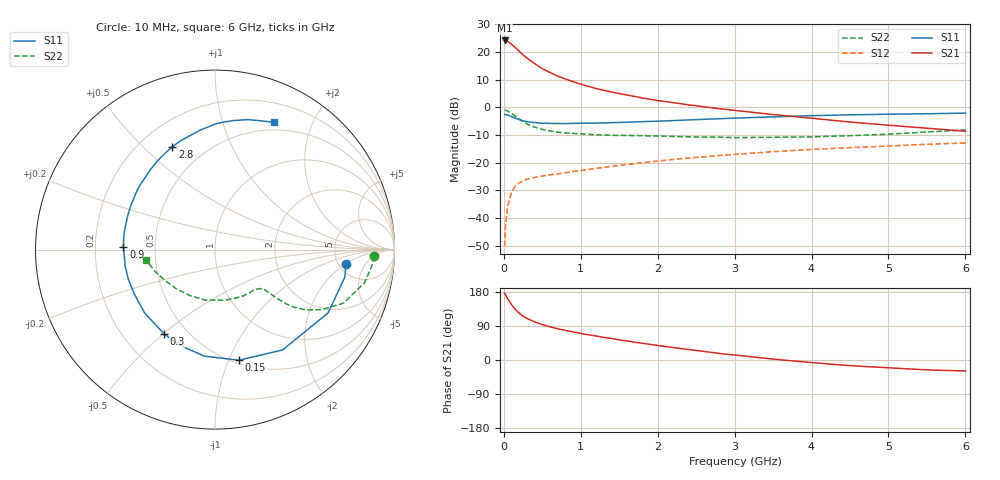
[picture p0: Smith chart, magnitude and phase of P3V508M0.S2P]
! SIEMENS Small Signal Semiconductors
! BFP181
! Si NPN RF Bipolar Junction Transistor in SOT143
! VCE = 0.5 V  IC = 8 mA
! Common Emitter S-Parameters:  March  1996
# GHz  S  MA  R  50
!  f  S11  S21  S12  S22
! GHz  MAG  ANG  MAG  ANG  MAG  ANG  MAG  ANG
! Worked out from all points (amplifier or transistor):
!   36 points, 10 MHz to 6 GHz, reference 50 ohm
!   highest |S21| = 24.1 dB at 10 MHz (marker M1)
!   |S21| within 3 dB of that: start of sweep to 165.1 MHz
!   unconditionally stable (mu >= 1): start of sweep to 10.12 MHz; 459.4 MHz to end of sweep
!   at 250 MHz: K = 0.61, MSG = 22.7 dB, |S12| = -26.6 dB
!   at 1.4 GHz: K = 1.95, MAG = 7.8 dB, |S12| = -21.3 dB
!   at 6 GHz: K = 2.00, MAG = -3.6 dB, |S12| = -12.9 dB
!   S11 on the Smith chart (normalised r, x): 10 MHz: 5.78, -2.06; 150 MHz: 0.53, -1.09; 300 MHz: 0.37, -0.50; 900 MHz: 0.32, +0.01; 2.8 GHz: 0.33, +0.62; 6 GHz: 0.41, +1.49
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0.01  0.7345 -6.4  16.03 176.4  0.0031 85.9  0.8855 -2.4
0.02  0.7391 -12.1  16.02 173.0  0.0067 80.3  0.8825 -5.1
0.05  0.7223 -29.2  15.46 161.7  0.0163 75.9  0.8534 -12.5
0.1  0.6742 -56.0  13.69 146.0  0.0292 61.7  0.7758 -22.6
0.15  0.6306 -77.7  11.87 133.3  0.0378 52.6  0.6829 -29.3
0.2  0.5966 -95.7  10.24 123.5  0.0432 46.8  0.6089 -33.5
0.25  0.5684 -110.1  8.793 115.8  0.0468 41.9  0.5464 -36.0
0.3  0.549 -121.2  7.711 110.0  0.0501 39.5  0.499 -37.3
0.4  0.5272 -138.3  6.111 100.5  0.0539 36.6  0.4378 -38.2
0.5  0.5134 -151.1  4.98 93.4  0.0573 35.0  0.3982 -38.5
0.6  0.5104 -161.1  4.235 87.5  0.0601 34.8  0.3721 -38.7
0.7  0.5089 -169.2  3.644 82.6  0.0625 35.3  0.3552 -39.0
0.9  0.5102 178.5  2.898 74.2  0.0692 36.1  0.3373 -40.3
1.1  0.5152 167.5  2.38 66.4  0.0754 37.1  0.3238 -42.6
1.5  0.5307 151.5  1.761 53.1  0.0888 38.1  0.3099 -48.6
1.8  0.5488 140.7  1.473 44.1  0.0993 37.9  0.3062 -54.5
2.2  0.5739 128.5  1.209 33.0  0.1138 36.5  0.2962 -63.7
2.8  0.6202 112.6  0.94 17.3  0.1343 33.2  0.2882 -79.3
3.5  0.669 97.5  0.737 2.4  0.1574 28.6  0.2865 -101.0
4.5  0.7271 81.7  0.54 -14.9  0.1861 20.1  0.306 -133.6
5.5  0.7623 70.2  0.418 -26.0  0.214 12.5  0.3571 -160.5
6  0.7818 65.0  0.368 -29.0  0.2263 8.1  0.3887 -171.5
